(* Logix 5000 AddOnInstructionDefinition export Generic_8PORT_IOL; software revision 20.03 *)

ADD_ON_INSTRUCTION Generic_8PORT_IOL   (* revision 1.0 *)
// Revision note:
// 4/27/17
VAR_OUTPUT
   Datastorage_Error : BOOL; {access Read Only, visible}
   Device_Not_Connected : BOOL; {access Read Only, visible}
   Invalid_Data : BOOL; {access Read Only, visible}
   IOL_Mode : BOOL; {access Read Only, visible}
END_VAR
VAR_IN_OUT
   PLC_Input : INT[223]; {required}
   PLC_Output : INT[151]; {required}
END_VAR
VAR_INPUT
   Port_Process_Data_Size : INT; {visible}
   Port_Number : INT; {visible}
END_VAR
VAR_OUTPUT
   Process_Data : INT; {access Read Only}
   Wrong_VID_DID : BOOL; {access Read Only, visible}
   IN_Data1 : INT; {visible}
   IN_Data2 : INT; {visible}
   IN_Data3 : INT; {visible}
   IN_Data4 : INT; {visible}
   Out_Data1 : INT; {visible}
   Out_Data2 : INT; {visible}
   Out_Data3 : INT; {visible}
   Out_Data4 : INT; {visible}
   Vendor_ID : INT; {access Read Only, visible}
   Device_ID : INT; {access Read Only, visible}
END_VAR
VAR
   Data_Size : INT; {access None}
   Offset_Address : INT; {access None}
   Offset_StatusFlgs : INT; {access None}
   Process_Offset : INT; {access None}
   Process_PDI : INT; {access None}
   RealPort_Num : INT; {access None}
   StatusFlgs_Offset : INT; {access None}
   Process_Out_Offset : INT; {access None}
END_VAR

ROUTINE Logic   (* ladder *)
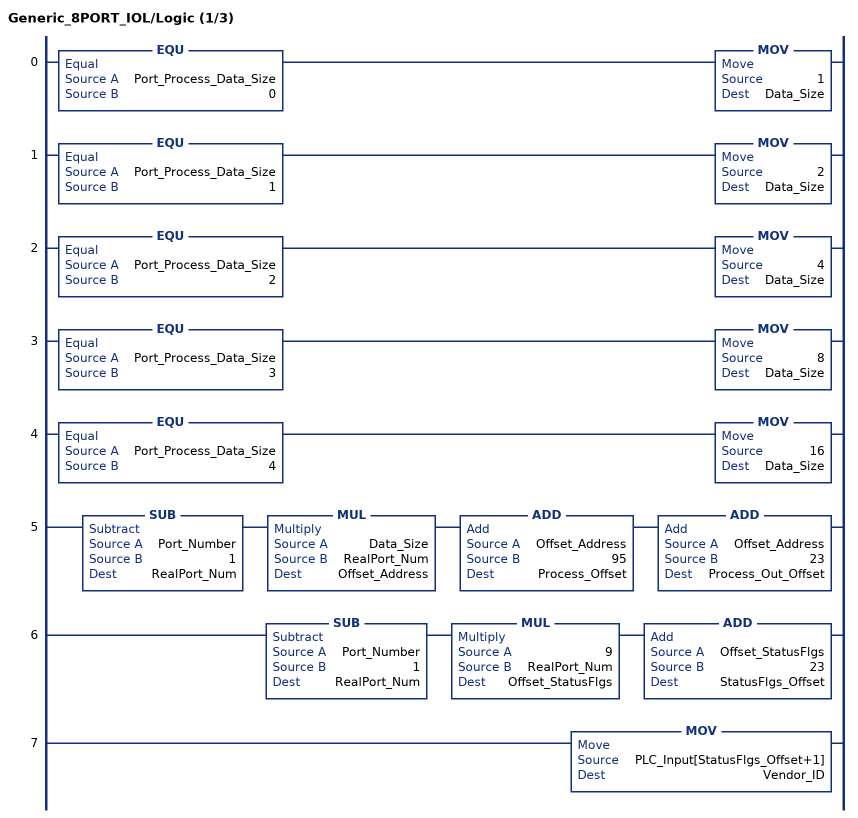
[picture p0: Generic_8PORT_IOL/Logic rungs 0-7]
   0: EQU(Port_Process_Data_Size,0)MOV(1,Data_Size);
   1: EQU(Port_Process_Data_Size,1)MOV(2,Data_Size);
   2: EQU(Port_Process_Data_Size,2)MOV(4,Data_Size);
   3: EQU(Port_Process_Data_Size,3)MOV(8,Data_Size);
   4: EQU(Port_Process_Data_Size,4)MOV(16,Data_Size);
   5: SUB(Port_Number,1,RealPort_Num)MUL(Data_Size,RealPort_Num,Offset_Address)ADD(Offset_Address,95,Process_Offset)ADD(Offset_Address,23,Process_Out_Offset);
   6: SUB(Port_Number,1,RealPort_Num)MUL(9,RealPort_Num,Offset_StatusFlgs)ADD(Offset_StatusFlgs,23,StatusFlgs_Offset);
   7: MOV(PLC_Input[StatusFlgs_Offset+1],Vendor_ID);
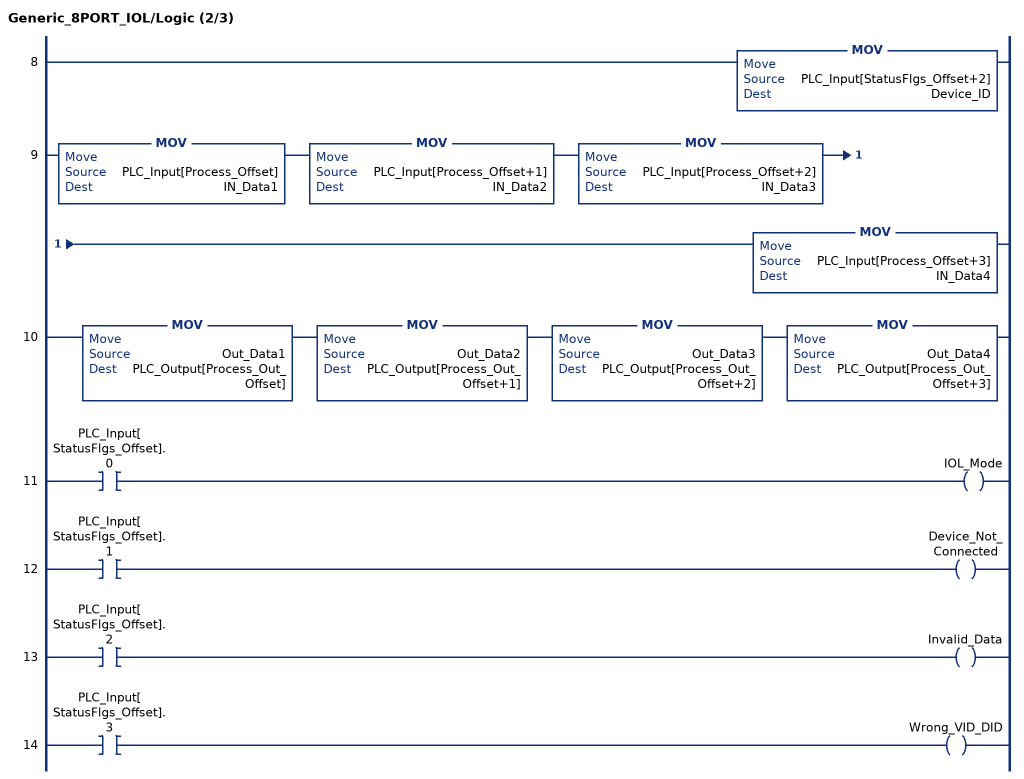
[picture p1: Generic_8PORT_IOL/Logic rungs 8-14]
   8: MOV(PLC_Input[StatusFlgs_Offset+2],Device_ID);
   9: MOV(PLC_Input[Process_Offset],IN_Data1)MOV(PLC_Input[Process_Offset+1],IN_Data2)MOV(PLC_Input[Process_Offset+2],IN_Data3)MOV(PLC_Input[Process_Offset+3],IN_Data4);
   10: MOV(Out_Data1,PLC_Output[Process_Out_Offset])MOV(Out_Data2,PLC_Output[Process_Out_Offset+1])MOV(Out_Data3,PLC_Output[Process_Out_Offset+2])MOV(Out_Data4,PLC_Output[Process_Out_Offset+3]);
   11: XIC(PLC_Input[StatusFlgs_Offset].0)OTE(IOL_Mode);
   12: XIC(PLC_Input[StatusFlgs_Offset].1)OTE(Device_Not_Connected);
   13: XIC(PLC_Input[StatusFlgs_Offset].2)OTE(Invalid_Data);
   14: XIC(PLC_Input[StatusFlgs_Offset].3)OTE(Wrong_VID_DID);
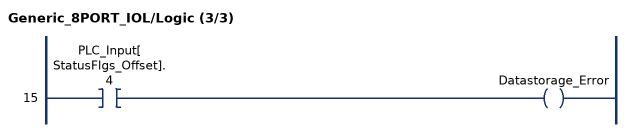
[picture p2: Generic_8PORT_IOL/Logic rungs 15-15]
   15: XIC(PLC_Input[StatusFlgs_Offset].4)OTE(Datastorage_Error);
END_ROUTINE
END_ADD_ON_INSTRUCTION
